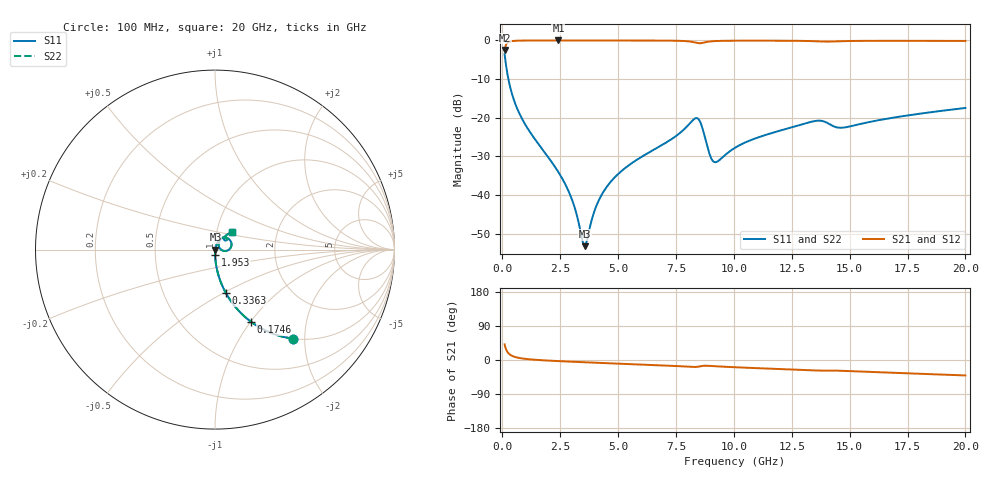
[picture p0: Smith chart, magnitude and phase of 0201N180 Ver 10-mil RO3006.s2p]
# GHz S MA R 50
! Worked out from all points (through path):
!   1601 points, 100 MHz to 20 GHz, reference 50 ohm
!   highest |S21| = -0.02 dB at 2.426 GHz (marker M1); lowest = -2.5 dB at 100 MHz (marker M2)
!   group delay of S21, straight-line fit = 6.27 ps
!   lowest |S11| = -53.2 dB at 3.558 GHz (marker M3), VSWR 1.00, Z = 50.2 - j0.0257 ohm
!   |S11| at or under -10 dB: 263 MHz to end of sweep
!   |S22| runs from -53.2 to -3.6 dB; largest |S21 - S12| = 0
!   S11 on the Smith chart (normalised r, x): 100 MHz: 1.00, -1.76; 174.6 MHz: 1.00, -1.01; 336.3 MHz: 1.00, -0.52; 1.953 GHz: 1.00, -0.06; 20 GHz: 1.18, +0.23
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0.1  0.6608 -48.7  0.7499 41.2  0.7499 41.2  0.6608 -48.7
0.174625  0.4497 -63.5  0.8925 26.4  0.8925 26.4  0.4497 -63.5
0.3363125  0.2514 -75.8  0.9671 14.0  0.9671 14.0  0.2514 -75.8
0.871125  0.09483 -85.4  0.9945 4.0  0.9945 4.0  0.09483 -85.4
1.953188  0.03184 -88.7  0.9979 -1.5  0.9979 -1.5  0.03184 -88.7
2.425813  0.01981 -87.8  0.998 -3.0  0.998 -3.0  0.01981 -87.8
3.010375  0.008758 -81.4  0.9979 -4.6  0.9979 -4.6  0.008758 -81.4
3.420812  0.002953 -49.1  0.9978 -5.6  0.9978 -5.6  0.002953 -49.1
3.557625  0.002195 -6.7  0.9977 -6.0  0.9977 -6.0  0.002195 -6.7
4.067563  0.007336 63.8  0.9975 -7.2  0.9975 -7.2  0.007336 63.8
4.565062  0.01348 70.5  0.9972 -8.4  0.9972 -8.4  0.01348 70.5
5.385937  0.02341 72.3  0.9966 -10.4  0.9966 -10.4  0.02341 72.3
6.741625  0.04185 70.1  0.9945 -13.7  0.9945 -13.7  0.04185 70.1
8.370938  0.09906 29.6  0.9306 -18.3  0.9306 -18.3  0.09906 29.6
8.569937  0.0852 4.9  0.9198 -16.1  0.9198 -16.1  0.0852 4.9
8.943062  0.0345 -1.3  0.9663 -15.5  0.9663 -15.5  0.0345 -1.3
9.129625  0.02708 18.8  0.9775 -16.2  0.9775 -16.2  0.02708 18.8
10.05  0.04099 59.0  0.9905 -19.1  0.9905 -19.1  0.04099 59.0
13.37081  0.08918 51.7  0.9788 -27.3  0.9788 -27.3  0.08918 51.7
14.65188  0.07439 45.6  0.9767 -28.5  0.9767 -28.5  0.07439 45.6
16.69162  0.09821 52.2  0.9872 -33.3  0.9872 -33.3  0.09821 52.2
20  0.134 46.5  0.984 -40.7  0.984 -40.7  0.134 46.5
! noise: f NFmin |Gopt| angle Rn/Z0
0.1  0.0005675  0.9247  0.3235  0.001671
2.301  0.003938  0.7702  3.922  0.003488
4.515  0.006761  0.7419  7.567  0.00523
6.729  0.01089  0.7593  11.22  0.00908
8.943  0.03452  0.8917  14.99  0.06828
11.14  0.01696  0.7471  18.51  0.01315
13.36  0.02963  0.82  22.19  0.03323
15.57  0.02504  0.7608  25.72  0.02019
17.79  0.02189  0.6997  29.08  0.01339
20  0.0227  0.6798  32.45  0.01268
